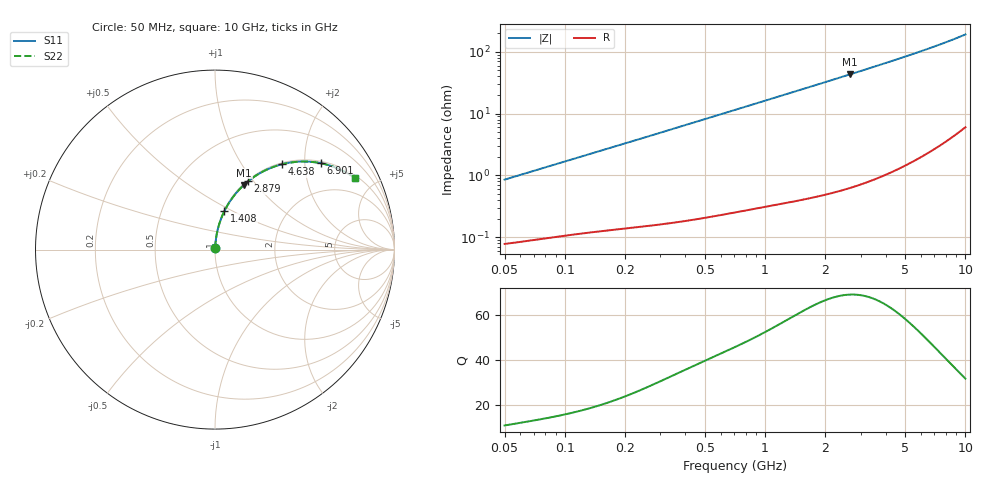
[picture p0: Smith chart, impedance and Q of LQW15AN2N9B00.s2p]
!Murata Part Number: LQW15AN2N9B00
!These Parameters are Measured in Series Mode Connection
!  o--[Z]--o
!Port1  Port2
!  o-------o
!Freq. Start=50[MHz] Stop=10[GHz], 401[Steps]
# Hz S RI R 50
!Freq.(Hz)	S 11(Real)	S 11(Imag)	S 21(Real)	S 21(Imag)	S 12(Real)	S 12(Imag)	S 22(Real)	S 22(Imag)
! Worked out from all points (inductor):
!   401 points, 50 MHz to 10 GHz, reference 50 ohm
!   read as one part in series: L = 2.7 nH near 51.34 MHz
!   highest Q = 68.9 at 2.659 GHz (marker M1), where L = 2.59 nH
!   S11 on the Smith chart (normalised r, x): 50 MHz: 1.00, +0.02; 1.408 GHz: 1.01, +0.46; 2.879 GHz: 1.01, +0.94; 4.638 GHz: 1.03, +1.54; 6.901 GHz: 1.05, +2.40; 10 GHz: 1.12, +3.82
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5e7  0.000851 0.00851  0.9991 -0.00851  0.9991 -0.00851  0.000851 0.00851
5.134228e7  0.000863 0.00873  0.9991 -0.00873  0.9991 -0.00873  0.000863 0.00873
1.214486e8  0.00155 0.0202  0.9984 -0.0202  0.9984 -0.0202  0.00155 0.0202
1.956524e8  0.0024 0.0321  0.9976 -0.0321  0.9976 -0.0321  0.0024 0.0321
2.949953e8  0.00392 0.0481  0.9961 -0.0481  0.9961 -0.0481  0.00392 0.0481
4.689809e8  0.00777 0.0757  0.9922 -0.0757  0.9922 -0.0757  0.00777 0.0757
7.071068e8  0.0154 0.1128  0.9846 -0.1128  0.9846 -0.1128  0.0154 0.1128
1.011124e9  0.029 0.1586  0.971 -0.1586  0.971 -0.1586  0.029 0.1586
1.408053e9  0.0527 0.2151  0.9473 -0.2151  0.9473 -0.2151  0.0527 0.2151
1.717543e9  0.0753 0.2561  0.9247 -0.2561  0.9247 -0.2561  0.0753 0.2561
2.151302e9  0.1122 0.3083  0.8878 -0.3083  0.8878 -0.3083  0.1122 0.3083
2.659148e9  0.1614 0.3607  0.8386 -0.3607  0.8386 -0.3607  0.1614 0.3607
2.879108e9  0.1841 0.3804  0.8159 -0.3804  0.8159 -0.3804  0.1841 0.3804
3.465724e9  0.2474 0.4241  0.7526 -0.4241  0.7526 -0.4241  0.2474 0.4241
4.171863e9  0.3251 0.4606  0.6749 -0.4606  0.6749 -0.4606  0.3251 0.4606
4.638213e9  0.3755 0.4761  0.6245 -0.4761  0.6245 -0.4761  0.3755 0.4761
5.657692e9  0.4791 0.4904  0.5209 -0.4904  0.5209 -0.4904  0.4791 0.4904
6.290134e9  0.5373 0.4887  0.4627 -0.4887  0.4627 -0.4887  0.5373 0.4887
6.901252e9  0.5884 0.4814  0.4116 -0.4814  0.4116 -0.4814  0.5884 0.4814
8.198065e9  0.681 0.4536  0.319 -0.4536  0.319 -0.4536  0.681 0.4536
9.48396e9  0.7535 0.4164  0.2465 -0.4164  0.2465 -0.4164  0.7535 0.4164
1e10  0.7779 0.4002  0.2221 -0.4002  0.2221 -0.4002  0.7779 0.4002
